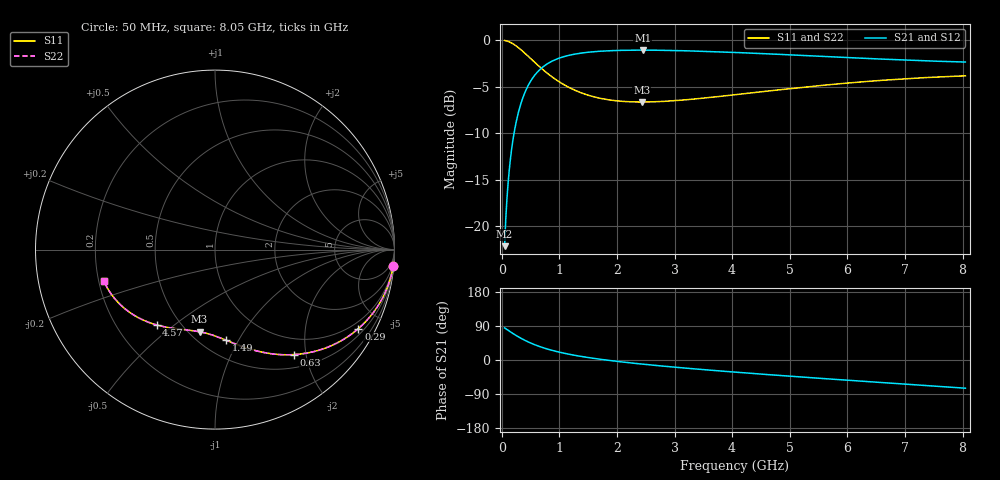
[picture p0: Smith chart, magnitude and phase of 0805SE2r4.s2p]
! AVX Thin Film Operation		Date: August 2001
! Description: Accu-P® Series, Thin Film, SMD, RF Capacitor
! Part Number: 08051J2R4ABT
! 50 MHz  -  8.05 GHz
! Serial Measurements
# mhz S db R 50
!	S11		S21		S12		S22
!	dB	Phase	dB	Phase	dB	Phase	dB	Phase
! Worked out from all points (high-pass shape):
!   401 points, 50 MHz to 8.05 GHz, reference 50 ohm
!   highest |S21| = -1.07 dB at 2.45 GHz (marker M1); lowest = -22.1 dB at 50 MHz (marker M2)
!   |S21| within 3 dB of the highest: 535.9 MHz to end of sweep
!   lowest |S11| = -6.6 dB at 2.43 GHz (marker M3), VSWR 2.74, Z = 28.2 - j33 ohm
!   |S11| at or under -10 dB: nowhere
!   |S22| runs from -6.6 to 0.0 dB; largest |S21 - S12| = 0
!   S11 on the Smith chart (normalised r, x): 50 MHz: 1, -22; 290 MHz: 0.72, -3.76; 630 MHz: 0.71, -1.79; 1.49 GHz: 0.65, -0.89; 4.57 GHz: 0.37, -0.43; 8.05 GHz: 0.22, -0.13
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50  -0.03 -5.3  -22.11 84.7  -22.11 84.7  -0.03 -5.3
70  -0.05 -7.4  -19.22 82.6  -19.22 82.6  -0.05 -7.4
110  -0.13 -11.6  -15.38 78.4  -15.38 78.4  -0.13 -11.6
150  -0.23 -15.6  -12.81 74.4  -12.81 74.4  -0.23 -15.6
210  -0.44 -21.5  -10.13 68.5  -10.13 68.5  -0.44 -21.5
290  -0.80 -28.9  -7.74 61.1  -7.74 61.1  -0.80 -28.9
450  -1.67 -41.6  -4.97 48.4  -4.97 48.4  -1.67 -41.6
630  -2.70 -52.9  -3.35 37.0  -3.35 37.0  -2.70 -53.0
790  -3.54 -60.9  -2.54 29.0  -2.54 29.0  -3.54 -61.0
970  -4.36 -68.2  -1.99 21.7  -1.99 21.7  -4.36 -68.2
1170  -5.08 -74.8  -1.62 15.2  -1.62 15.2  -5.08 -74.8
1390  -5.67 -80.8  -1.38 9.2  -1.38 9.2  -5.67 -80.8
1490  -5.88 -83.2  -1.30 6.7  -1.30 6.7  -5.88 -83.2
1910  -6.45 -91.9  -1.12 -2.0  -1.12 -2.0  -6.45 -91.9
2430  -6.64 -100.6  -1.07 -10.7  -1.07 -10.7  -6.64 -100.7
2450  -6.64 -100.9  -1.07 -11.0  -1.07 -11.0  -6.64 -101.0
2730  -6.59 -105.1  -1.08 -15.1  -1.08 -15.1  -6.59 -105.1
4050  -5.85 -121.9  -1.31 -32.0  -1.31 -32.0  -5.85 -121.9
4570  -5.49 -127.8  -1.45 -38.0  -1.45 -38.0  -5.49 -127.9
5390  -4.96 -136.8  -1.68 -46.9  -1.68 -46.9  -4.96 -136.8
6730  -4.25 -150.7  -2.06 -60.9  -2.06 -60.9  -4.25 -150.8
8050  -3.83 -164.3  -2.35 -74.4  -2.35 -74.4  -3.83 -164.3
